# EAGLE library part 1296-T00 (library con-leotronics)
1.27mm SINGLE ROW FEMALE SOCKET Source: http://www.leotronics.co.uk/Conexcon/Data%20Sheets/sec.%20A/1296ing.pdf
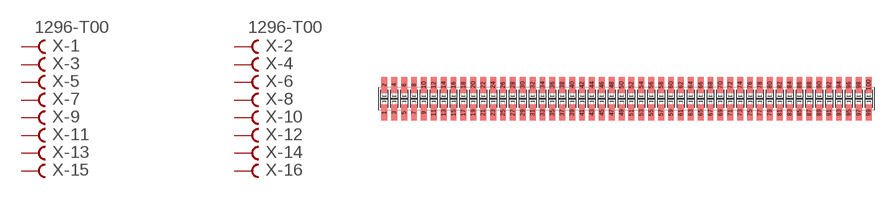
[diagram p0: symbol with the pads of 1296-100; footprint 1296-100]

Designator prefix X; gates -1=FVAL -2=FVAL -3=F -4=F -5=F -6=F -7=F -8=F -9=F -10=F -11=F -12=F -13=F -14=F -15=F -16=F -17=F -18=F -19=F -20=F -21=F -22=F -23=F -24=F -25=F -26=F -27=F -28=F -29=F -30=F -31=F -32=F -33=F -34=F -35=F -36=F -37=F -38=F -39=F -40=F -41=F -42=F -43=F -44=F -45=F -46=F -47=F -48=F -49=F -50=F -51=F -52=F -53=F -54=F -55=F -56=F -57=F -58=F -59=F -60=F -61=F -62=F -63=F -64=F -65=F -66=F -67=F -68=F -69=F -70=F -71=F -72=F -73=F -74=F -75=F -76=F -77=F -78=F -79=F -80=F -81=F -82=F -83=F -84=F -85=F -86=F -87=F -88=F -89=F -90=F -91=F -92=F -93=F -94=F -95=F -96=F -97=F -98=F -99=F -100=F

## 1296-T00 (OC_FARNELL: unknown; OC_NEWARK: unknown)  [1296-100]
1  -1:B  pas
2  -2:B  pas
3  -3:B  pas
4  -4:B  pas
5  -5:B  pas
6  -6:B  pas
7  -7:B  pas
8  -8:B  pas
9  -9:B  pas
10  -10:B  pas
11  -11:B  pas
12  -12:B  pas
13  -13:B  pas
14  -14:B  pas
15  -15:B  pas
16  -16:B  pas
17  -17:B  pas
18  -18:B  pas
19  -19:B  pas
20  -20:B  pas
21  -21:B  pas
22  -22:B  pas
23  -23:B  pas
24  -24:B  pas
25  -25:B  pas
26  -26:B  pas
27  -27:B  pas
28  -28:B  pas
29  -29:B  pas
30  -30:B  pas
31  -31:B  pas
32  -32:B  pas
33  -33:B  pas
34  -34:B  pas
35  -35:B  pas
36  -36:B  pas
37  -37:B  pas
38  -38:B  pas
39  -39:B  pas
40  -40:B  pas
41  -41:B  pas
42  -42:B  pas
43  -43:B  pas
44  -44:B  pas
45  -45:B  pas
46  -46:B  pas
47  -47:B  pas
48  -48:B  pas
49  -49:B  pas
50  -50:B  pas
51  -51:B  pas
52  -52:B  pas
53  -53:B  pas
54  -54:B  pas
55  -55:B  pas
56  -56:B  pas
57  -57:B  pas
58  -58:B  pas
59  -59:B  pas
60  -60:B  pas
61  -61:B  pas
62  -62:B  pas
63  -63:B  pas
64  -64:B  pas
65  -65:B  pas
66  -66:B  pas
67  -67:B  pas
68  -68:B  pas
69  -69:B  pas
70  -70:B  pas
71  -71:B  pas
72  -72:B  pas
73  -73:B  pas
74  -74:B  pas
75  -75:B  pas
76  -76:B  pas
77  -77:B  pas
78  -78:B  pas
79  -79:B  pas
80  -80:B  pas
81  -81:B  pas
82  -82:B  pas
83  -83:B  pas
84  -84:B  pas
85  -85:B  pas
86  -86:B  pas
87  -87:B  pas
88  -88:B  pas
89  -89:B  pas
90  -90:B  pas
91  -91:B  pas
92  -92:B  pas
93  -93:B  pas
94  -94:B  pas
95  -95:B  pas
96  -96:B  pas
97  -97:B  pas
98  -98:B  pas
99  -99:B  pas
100  -100:B  pas

## Footprint 1296-100 (pad centres in mm)
1.27mm SINGLE ROW FEMALE SOCKET Source: http://www.leotronics.co.uk/Conexcon/Data%20Sheets/sec.%20A/1296ing.pdf
smd 0.76 x 2.05: 1 -31.115,-1.78; 2 -31.115,1.78; 3 -29.845,-1.78; 4 -29.845,1.78; 5 -28.575,-1.78; 6 -28.575,1.78; 7 -27.305,-1.78; 8 -27.305,1.78; 9 -26.035,-1.78; 10 -26.035,1.78; 11 -24.765,-1.78; 12 -24.765,1.78; 13 -23.495,-1.78; 14 -23.495,1.78; 15 -22.225,-1.78; 16 -22.225,1.78; 17 -20.955,-1.78; 18 -20.955,1.78; 19 -19.685,-1.78; 20 -19.685,1.78; 21 -18.415,-1.78; 22 -18.415,1.78; 23 -17.145,-1.78; 24 -17.145,1.78; 25 -15.875,-1.78; 26 -15.875,1.78; 27 -14.605,-1.78; 28 -14.605,1.78; 29 -13.335,-1.78; 30 -13.335,1.78; 31 -12.065,-1.78; 32 -12.065,1.78; 33 -10.795,-1.78; 34 -10.795,1.78; 35 -9.525,-1.78; 36 -9.525,1.78; 37 -8.255,-1.78; 38 -8.255,1.78; 39 -6.985,-1.78; 40 -6.985,1.78; 41 -5.715,-1.78; 42 -5.715,1.78; 43 -4.445,-1.78; 44 -4.445,1.78; 45 -3.175,-1.78; 46 -3.175,1.78; 47 -1.905,-1.78; 48 -1.905,1.78; 49 -0.635,-1.78; 50 -0.635,1.78; 51 0.635,-1.78; 52 0.635,1.78; 53 1.905,-1.78; 54 1.905,1.78; 55 3.175,-1.78; 56 3.175,1.78; 57 4.445,-1.78; 58 4.445,1.78; 59 5.715,-1.78; 60 5.715,1.78; 61 6.985,-1.78; 62 6.985,1.78; 63 8.255,-1.78; 64 8.255,1.78; 65 9.525,-1.78; 66 9.525,1.78; 67 10.795,-1.78; 68 10.795,1.78; 69 12.065,-1.78; 70 12.065,1.78; 71 13.335,-1.78; 72 13.335,1.78; 73 14.605,-1.78; 74 14.605,1.78; 75 15.875,-1.78; 76 15.875,1.78; 77 17.145,-1.78; 78 17.145,1.78; 79 18.415,-1.78; 80 18.415,1.78; 81 19.685,-1.78; 82 19.685,1.78; 83 20.955,-1.78; 84 20.955,1.78; 85 22.225,-1.78; 86 22.225,1.78; 87 23.495,-1.78; 88 23.495,1.78; 89 24.765,-1.78; 90 24.765,1.78; 91 26.035,-1.78; 92 26.035,1.78; 93 27.305,-1.78; 94 27.305,1.78; 95 28.575,-1.78; 96 28.575,1.78; 97 29.845,-1.78; 98 29.845,1.78; 99 31.115,-1.78; 100 31.115,1.78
